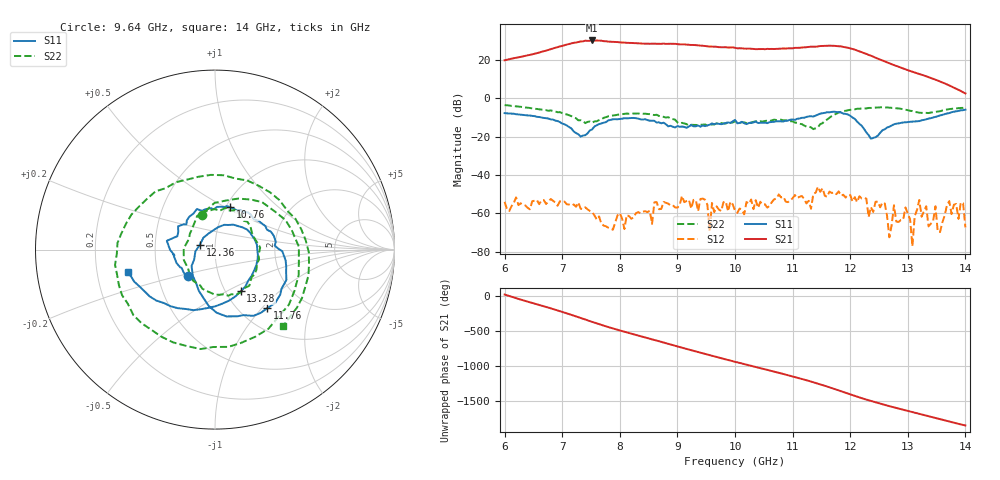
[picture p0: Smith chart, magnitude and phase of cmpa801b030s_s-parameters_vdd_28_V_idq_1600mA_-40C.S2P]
!Keysight Technologies,E5071C,MY46110325,B.14.03
!Date: Tue Aug 11 10:37:03 2020
!Data & Calibration Information:
!Freq	S11:SOLT2(ON)	S21:SOLT2(ON)	S12:SOLT2(ON)	S22:SOLT2(ON)
!PortZ  Port1:50+j0  Port2:50+j0
!Above PortZ is port z conversion or system Z0 setting when saving the data.
!When reading, reference impedance value at option line is always used.
# Hz S dB R 50
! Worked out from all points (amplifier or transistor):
!   201 points, 6 GHz to 14 GHz, reference 50 ohm
!   highest |S21| = 30.1 dB at 7.52 GHz (marker M1)
!   |S21| within 3 dB of that: 6.976 GHz to 9.501 GHz (2.526 GHz wide, 30.7 % of centre)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
!   unconditionally stable (mu >= 1): start of sweep to end of sweep
!   at 7.32 GHz: K = 11.49, MAG = 30.0 dB, |S12| = -57.5 dB
!   at 10 GHz: K = 17.94, MAG = 26.9 dB, |S12| = -58.6 dB
!   at 14 GHz: K = 433.51, MAG = 5.5 dB, |S12| = -67.3 dB
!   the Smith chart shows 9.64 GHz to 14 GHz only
!   S11 on the Smith chart (normalised r, x): 9.64 GHz: 0.71, -0.22; 10.76 GHz: 1.05, +0.53; 11.76 GHz: 1.32, -1.07; 12.36 GHz: 0.84, +0.05; 13.28 GHz: 1.18, -0.59; 14 GHz: 0.34, -0.11
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6e9  -7.74 -37.2  19.80 19.7  -53.93 167.8  -3.57 -28.1
6.48e9  -9.19 -89.6  22.88 -101.1  -53.67 95.0  -5.25 -116.4
6.88e9  -11.63 -138.8  26.32 162.0  -54.30 18.6  -6.92 159.3
7.16e9  -15.77 -164.8  28.57 88.6  -55.87 -33.7  -9.32 110.2
7.36e9  -19.40 -135.8  29.65 32.7  -57.77 -80.9  -11.75 92.0
7.52e9  -16.21 -127.3  30.12 -12.1  -59.28 -98.0  -12.79 91.5
7.8e9  -11.57 -154.3  29.52 -86.5  -67.43 146.9  -9.39 67.3
8.16e9  -10.38 153.2  28.87 -171.9  -61.39 11.6  -8.06 20.1
8.68e9  -12.52 77.5  28.39 69.9  -57.78 -87.8  -9.22 -52.3
9.08e9  -14.72 -21.9  28.09 -21.6  -50.90 164.4  -12.79 -125.7
9.32e9  -14.62 -79.3  27.68 -76.8  -53.09 92.3  -13.89 170.7
9.64e9  -13.59 -135.2  26.86 -146.5  -59.31 46.4  -13.62 110.5
1e10  -11.28 169.6  26.30 135.2  -58.60 -90.0  -11.99 61.2
1.076e10  -12.02 69.9  25.77 -21.5  -50.10 170.3  -11.13 -58.6
1.108e10  -10.70 33.4  26.29 -91.5  -51.97 120.2  -12.80 -107.8
1.136e10  -9.54 3.8  26.84 -157.8  -49.69 80.1  -16.08 158.1
1.176e10  -7.19 -48.5  27.19 97.4  -49.96 -41.3  -8.06 32.4
1.204e10  -10.02 -96.4  25.69 17.9  -53.79 -114.4  -5.79 -36.6
1.236e10  -21.06 162.1  22.19 -65.5  -56.67 171.6  -5.04 -106.4
1.268e10  -14.82 46.8  18.19 -139.4  -72.46 57.9  -4.87 -159.7
1.328e10  -11.27 -58.3  11.89 93.0  -58.76 82.4  -7.60 93.1
1.4e10  -5.96 -165.5  2.53 -56.0  -67.26 -71.6  -4.87 -48.4
